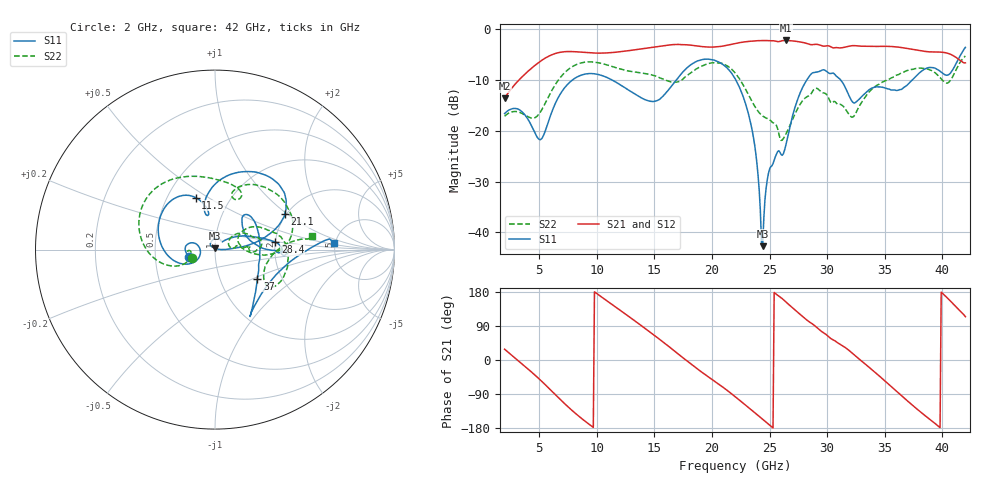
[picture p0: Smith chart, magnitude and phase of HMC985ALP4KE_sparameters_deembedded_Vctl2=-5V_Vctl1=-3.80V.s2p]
!s2p File: Measurements: S11, S21, S12, S22
# GHz S dB R 50.0
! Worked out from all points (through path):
!   401 points, 2 GHz to 42 GHz, reference 50 ohm
!   highest |S21| = -2.20 dB at 26.4 GHz (marker M1); lowest = -13.6 dB at 2 GHz (marker M2)
!   lowest |S11| = -42.7 dB at 24.4 GHz (marker M3), VSWR 1.01, Z = 49.8 + j0.706 ohm
!   |S11| at or under -10 dB: start of sweep to 7.882 GHz; 22.07 GHz to 28.23 GHz (6.153 GHz wide, 24.5 % of centre); 31.18 GHz to 37.38 GHz (6.202 GHz wide, 18.1 % of centre)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
!   |S22| runs from -21.9 to -5.3 dB; largest |S21 - S12| = 0.001
!   S11 on the Smith chart (normalised r, x): 2 GHz: 0.75, -0.06; 11.5 GHz: 0.69, +0.44; 21.1 GHz: 1.96, +0.96; 28.4 GHz: 2.00, +0.19; 37 GHz: 1.50, -0.53; 42 GHz: 4.86, +0.68
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2  -16.59 -164.7  -13.60 28.5  -13.60 28.5  -17.12 -160.0
5.1  -21.74 -172.9  -6.31 -52.8  -6.31 -52.8  -16.31 -159.1
6.3  -15.13 -152.5  -4.84 -88.3  -4.84 -88.3  -11.26 -161.2
8.7  -9.00 149.4  -4.52 -154.7  -4.52 -154.7  -6.59 151.6
11.5  -10.20 110.4  -4.55 142.8  -4.55 142.8  -7.45 105.7
13.6  -13.15 100.3  -3.94 96.6  -3.94 96.7  -8.51 76.9
15.4  -13.87 104.7  -3.35 55.8  -3.35 55.8  -9.47 63.7
17.9  -7.45 79.1  -3.07 -4.1  -3.07 -4.1  -9.00 71.4
21.1  -7.19 27.0  -3.23 -75.1  -3.23 -75.1  -6.94 15.7
22  -9.69 16.8  -2.81 -96.4  -2.81 -96.4  -8.56 0.6
23.5  -20.01 3.6  -2.32 -133.7  -2.32 -133.7  -14.30 -4.2
24.4  -42.71 104.6  -2.22 -156.4  -2.21 -156.3  -17.07 7.4
25  -27.53 128.9  -2.25 -171.6  -2.25 -171.6  -17.79 10.3
26.4  -22.94 44.3  -2.20 153.6  -2.20 153.7  -20.72 32.3
28.4  -9.41 7.1  -2.90 101.6  -2.90 101.7  -13.11 18.3
28.7  -8.62 2.0  -3.03 95.5  -3.03 95.5  -12.34 16.7
30.7  -8.98 -2.9  -3.62 50.2  -3.62 50.2  -14.28 3.1
32.4  -14.50 30.0  -3.22 12.3  -3.22 12.3  -16.86 26.8
35.4  -11.80 17.5  -3.37 -65.7  -3.37 -65.6  -9.79 18.7
37  -10.87 -34.5  -3.79 -108.7  -3.79 -108.6  -8.10 4.5
39.8  -8.26 -55.9  -4.49 -178.5  -4.49 -178.4  -9.49 -33.5
42  -3.55 3.4  -6.61 114.2  -6.61 114.3  -5.25 8.3
